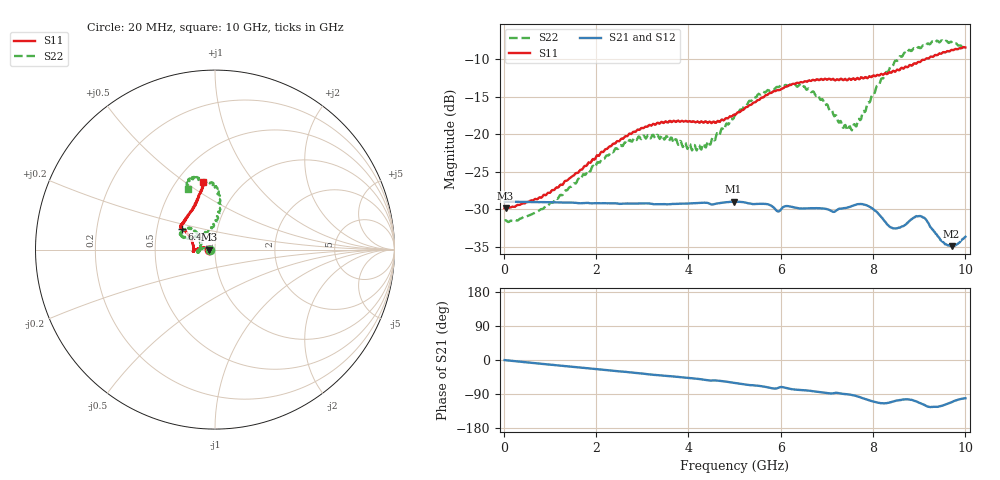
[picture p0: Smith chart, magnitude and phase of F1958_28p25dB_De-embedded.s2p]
! Integrated Device Technology
! Corporate Headquarters
! 6024 Silver Creek Valley Road
! San Jose, CA 95138  USA
! Phone:  1-408-284-8200
! Toll Free:  1-800-223-1366
! Webpage:  http://www.idt.com/
! Timing and RF Division
! 515 Groton Road, Suite 102
! Westford, MA 01886-6024
! Device:  F1958
! Description: 7-bit 0.25 dB Digital Step Attenuator
! Frequency:  0.001 -  6.000 GHz
! Package:  4x4 mm Thin QFN Plastic Package: 24 pin
! Ports:  2 RF, 12 DC
!  Pin  1  = D0
!  Pin  2  = VDD
!  Pin  3  = VMODE
!  Pin  4  = GND
!  Pin  5  = RF1  =  Port 1
!  Pin  6  = GND
!  Pin  7  = GND
!  Pin  8  = GND
!  Pin  9  = GND
!  Pin 10  = GND
!  Pin 11  = GND
!  Pin 12  = GND
!  Pin 13  = GND
!  Pin 14  = RF2  =  Port 2
!  Pin 15  = GND
!  Pin 16  = LE
!  Pin 17  = CLK
!  Pin 18  = DATA
!  Pin 19  = D6
!  Pin 20  = D5
!  Pin 21  = D4
!  Pin 22  = D3
!  Pin 23  = D2
!  Pin 24  = D1
! State:  113
! Atten State:  28.25 dB
! Voltage:  +3.30 Volts
! Current:  0.258 mA
! Data:  The device was measured on a F1958 evaluation board which has
!  individual transmission lines to the RF pins.  Data was collected
!  using a calibrated network analyzer.  The evaluation board was
!  de-embedded using Automatic Fixture Removal (AFR).
!  The reference plane is the edge of the package pin.
! Misc:
!  Action Tracker AT0419
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# GHz S dB R 50
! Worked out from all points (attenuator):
!   500 points, 20 MHz to 10 GHz, reference 50 ohm
!   highest |S21| = -29.01 dB at 4.98 GHz (marker M1); lowest = -34.9 dB at 9.7 GHz (marker M2)
!   lowest |S11| = -29.9 dB at 40 MHz (marker M3), VSWR 1.07, Z = 46.9 - j0.042 ohm
!   |S11| at or under -10 dB: start of sweep to 9.13 GHz
!   |S22| runs from -31.7 to -7.5 dB; largest |S21 - S12| = 0.00029
!   S11 on the Smith chart (normalised r, x): 20 MHz: 0.94, -0.00; 6.4 GHz: 0.67, +0.17; 10 GHz: 0.67, +0.59
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0.02  -29.88 -178.9  -29.04 -0.3  -29.03 -0.2  -31.52 -179.0
0.04  -29.91 -179.2  -29.02 -0.5  -29.01 -0.4  -31.49 -178.5
0.84  -28.32 171.0  -29.07 -10.3  -29.06 -10.3  -29.99 171.9
1.7  -24.70 170.9  -29.20 -20.4  -29.19 -20.3  -25.61 170.7
2.62  -20.33 176.9  -29.26 -31.1  -29.24 -31.2  -21.09 179.8
3.36  -18.56 -175.8  -29.34 -40.1  -29.35 -40.3  -20.43 -170.1
4.24  -18.46 -179.1  -29.17 -50.3  -29.18 -50.4  -21.51 168.1
4.98  -17.40 161.7  -29.01 -60.0  -29.02 -59.9  -17.87 137.3
5.02  -17.38 160.7  -29.01 -60.7  -29.02 -60.7  -17.31 137.8
5.6  -15.10 150.7  -29.30 -69.5  -29.31 -69.5  -14.40 139.9
5.94  -14.10 148.3  -30.32 -73.8  -30.34 -73.8  -13.69 148.3
6.4  -13.15 147.8  -29.90 -79.0  -29.92 -78.9  -13.41 155.4
6.68  -12.79 146.6  -29.87 -81.9  -29.90 -81.8  -14.34 157.3
7.5  -12.61 138.2  -29.70 -91.4  -29.70 -91.2  -18.95 119.4
7.68  -12.57 135.3  -29.33 -96.7  -29.32 -96.7  -17.99 99.3
7.9  -12.37 128.9  -29.59 -105.6  -29.58 -105.7  -15.71 89.1
8.34  -11.74 118.9  -32.23 -112.9  -32.23 -112.9  -11.51 83.9
8.66  -11.25 113.1  -32.25 -104.2  -32.25 -104.1  -9.28 87.7
9.04  -10.25 106.8  -30.97 -114.8  -30.98 -115.0  -8.47 97.4
9.5  -9.12 101.3  -34.35 -120.6  -34.34 -120.8  -7.49 108.8
9.7  -8.73 100.5  -34.95 -111.4  -34.95 -111.3  -7.66 111.9
10  -8.41 99.7  -33.69 -101.0  -33.71 -101.0  -8.60 113.9
